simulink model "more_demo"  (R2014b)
settings: Solver=ode45  StartTime=0.0  StopTime=10.0  RelTol=1e-3

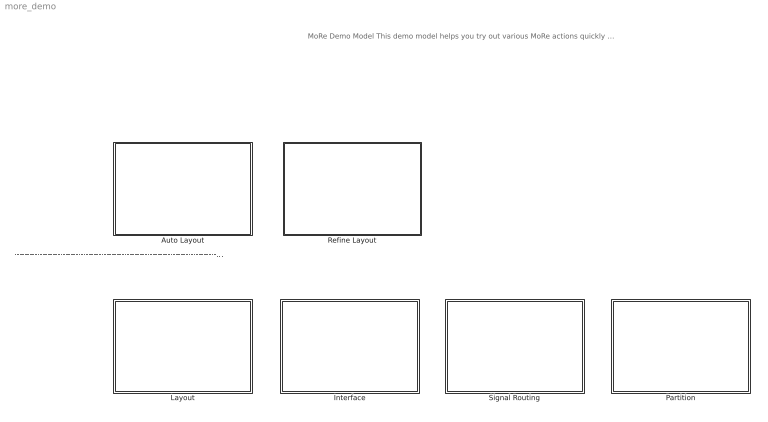
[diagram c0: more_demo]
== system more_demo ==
  note: -----------------------------------------------------------------------------------------------------------------------------------------------------------------
  note: MoRe Demo Model This demo model helps you try out various MoRe actions quickly and easily. To try out an action, navigate to the desired action via the corresponding category. The categories correspond to the MoRe menu. Please note: Demo models are not currently available for all MoRe actions.
  Auto Layout : Subsystem
  Interface : Subsystem
  Layout : Subsystem
  Partition : Subsystem
  Refine Layout : Subsystem
  Signal Routing : Subsystem

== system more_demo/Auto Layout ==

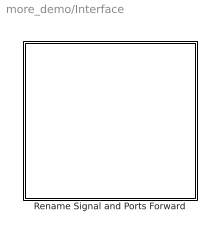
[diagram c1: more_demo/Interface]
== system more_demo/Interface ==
  Rename Signal and Ports Forward : Subsystem

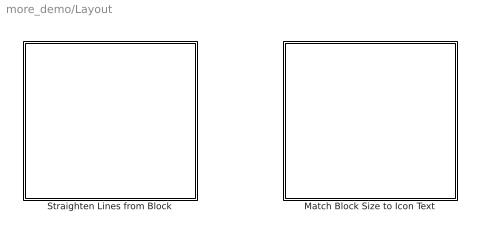
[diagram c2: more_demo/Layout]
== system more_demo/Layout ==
  Match Block Size to Icon Text : Subsystem
  Straighten Lines from Block : Subsystem

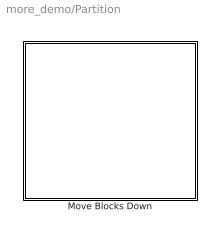
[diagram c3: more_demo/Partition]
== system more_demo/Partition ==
  Move Blocks Down : Subsystem

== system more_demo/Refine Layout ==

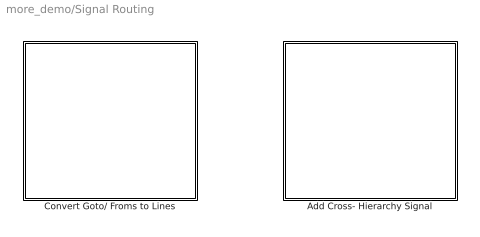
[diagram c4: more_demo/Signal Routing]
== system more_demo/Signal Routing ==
  Add Cross- Hierarchy Signal : Subsystem
  Convert Goto/ Froms to Lines : Subsystem

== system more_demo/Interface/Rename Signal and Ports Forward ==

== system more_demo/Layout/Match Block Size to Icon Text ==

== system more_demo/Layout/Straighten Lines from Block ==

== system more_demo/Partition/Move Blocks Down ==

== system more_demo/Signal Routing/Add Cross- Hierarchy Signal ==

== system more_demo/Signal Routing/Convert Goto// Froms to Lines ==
